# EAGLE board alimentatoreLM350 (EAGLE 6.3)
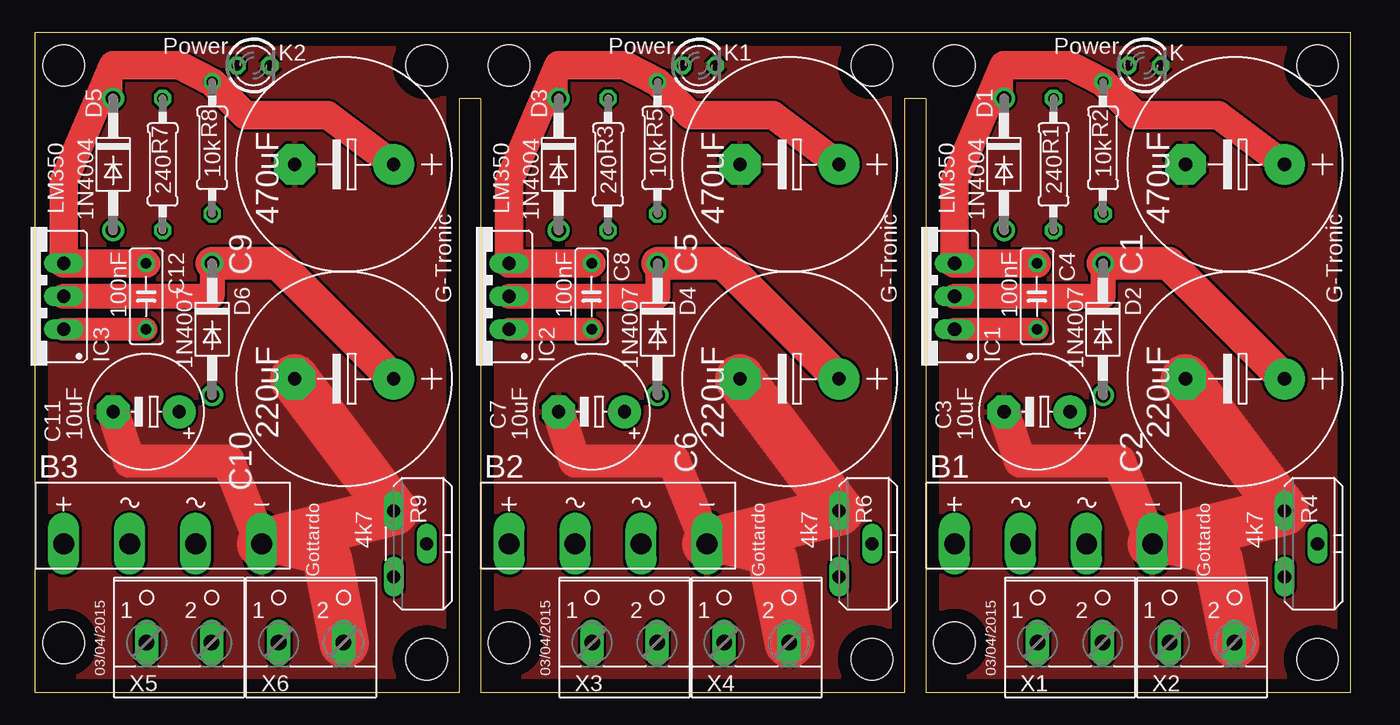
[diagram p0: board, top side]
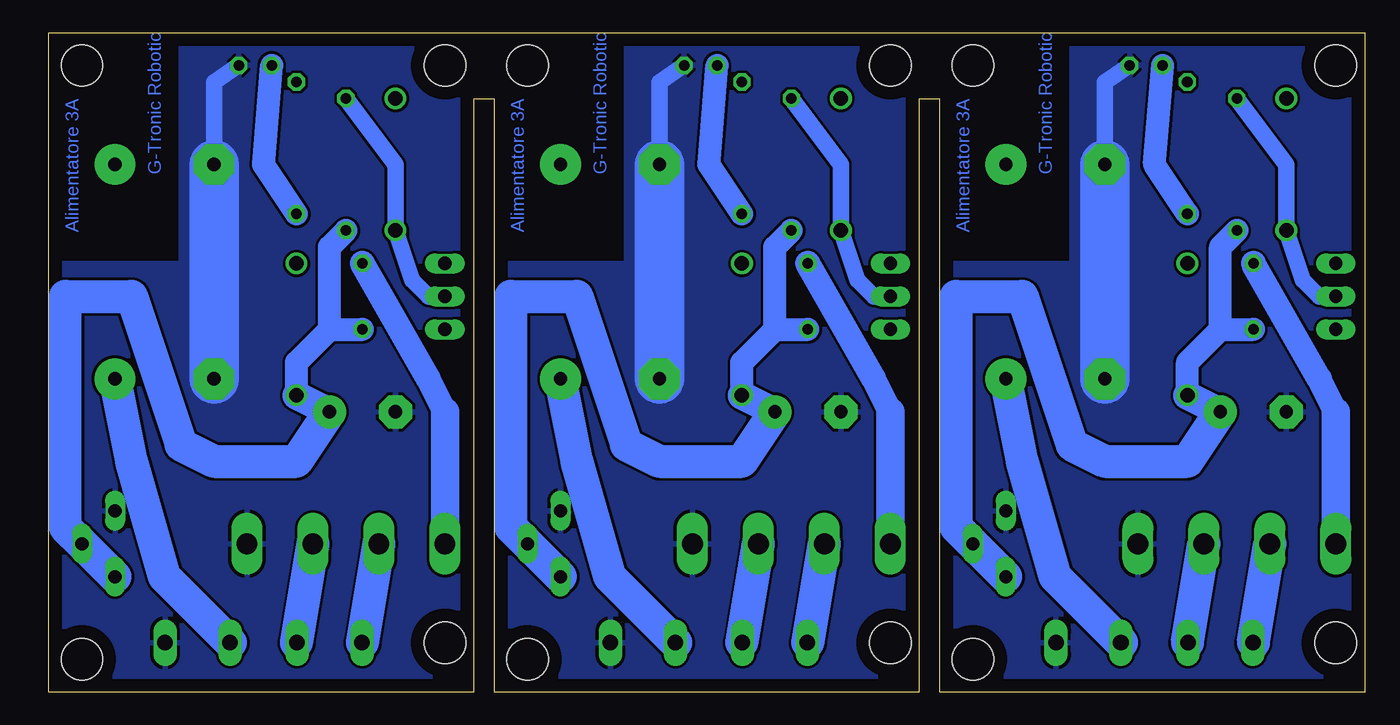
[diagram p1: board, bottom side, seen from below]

Size 101.27 x 50.78 mm. Coordinates in mm from the lower left corner, seen from the top.
Outline: 66.98,50.78 64.44,50.78
Outline: 101.27,0 101.27,50.78 0,50.78 0,0 32.69,0 32.69,45.7 34.29,45.7 34.29,0 66.98,0 66.98,45.7 68.58,45.7 68.58,0 101.27,0
Copper layers (1*16): Top 0.035mm / dielectric 1.5mm / Bottom 0.035mm
Design rules "default": minimum track width 10mil, minimum drill 24mil, track to track 8mil, track to pad 8mil, pad to pad 8mil, via to via 8mil, smd to smd 8mil, copper to edge 40mil, drill to drill 8mil, minimum pad ring 10mil, minimum via ring 8mil, stop-mask expansion 4mil, vias tented up to drill 0mil, thermal gap 10mil
Holes 3.2 mm at 70.79,3.81 98.73,2.54 70.79,48.26 98.73,48.26 36.5,3.81 64.44,2.54 36.5,48.26 64.44,48.26 2.21,3.81 30.15,2.54 2.21,48.26 30.15,48.26

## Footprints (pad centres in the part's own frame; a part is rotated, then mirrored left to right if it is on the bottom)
KBL = drill 1.6 long: + -7.62,-1.27; - 7.62,-1.27; AC1 2.54,-1.27; AC2 -2.54,-1.27
E7,5-16 = drill 1.016 pad 3.15: + -3.81,0 | drill 1.016 pad 3.15 octagon: - 3.81,0
E5-8,5 = drill 1.016 pad 2.54: + -2.54,0 | drill 1.016 pad 2.54 octagon: - 2.54,0
C050-025X075 = drill 0.813 octagon: 1 -2.54,0; 2 2.54,0
DO41-10 = drill 1.118: A 5.08,0; C -5.08,0
317TS = drill 1.016 long: 1 -2.54,-2.54; 2 0,-2.54; 3 2.54,-2.54
LED3MM = drill 0.813 octagon: A -1.27,0; K 1.27,0
0207/10 = drill 0.813 octagon: 1 -5.08,0; 2 5.08,0
PT-10S = drill 1.016 long: A -2.54,-1.27; E 2.54,-1.27; S 0,1.27
W237-102 = drill 1.194 long: 1 -2.5,-1.27; 2 2.5,-1.27

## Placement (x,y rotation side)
B1  [KBL]  78.41,12.7 0 top
B2  [KBL]  44.12,12.7 0 top
B3  [KBL]  9.83,12.7 0 top
C1  470uF  [E7,5-16]  92.38,40.64 180 top
C2  220uF  [E7,5-16]  92.38,24.13 180 top
C3  10uF  [E5-8,5]  77.14,21.59 180 top
C4  100nF  [C050-025X075]  77.14,30.48 270 top
C5  470uF  [E7,5-16]  58.09,40.64 180 top
C6  220uF  [E7,5-16]  58.09,24.13 180 top
C7  10uF  [E5-8,5]  42.85,21.59 180 top
C8  100nF  [C050-025X075]  42.85,30.48 270 top
C9  470uF  [E7,5-16]  23.8,40.64 180 top
C10  220uF  [E7,5-16]  23.8,24.13 180 top
C11  10uF  [E5-8,5]  8.56,21.59 180 top
C12  100nF  [C050-025X075]  8.56,30.48 270 top
D1  1N4004  [DO41-10]  74.6,40.64 270 top
D2  1N4007  [DO41-10]  82.22,27.94 270 top
D3  1N4004  [DO41-10]  40.31,40.64 270 top
D4  1N4007  [DO41-10]  47.93,27.94 270 top
D5  1N4004  [DO41-10]  6.02,40.64 270 top
D6  1N4007  [DO41-10]  13.64,27.94 270 top
IC1  LM350  [317TS]  68.25,30.48 90 top
IC2  LM350  [317TS]  33.96,30.48 90 top
IC3  LM350  [317TS]  -0.33,30.48 90 top
K  Power  [LED3MM]  85.39,48.26 0 top
K1  Power  [LED3MM]  51.11,48.26 0 top
K2  Power  [LED3MM]  16.82,48.26 0 top
R1  240  [0207/10]  78.41,40.64 90 top
R2  10k  [0207/10]  82.22,41.91 90 top
R3  240  [0207/10]  44.12,40.64 90 top
R4  4k7  [PT-10S]  97.46,11.43 270 top
R5  10k  [0207/10]  47.93,41.91 90 top
R6  4k7  [PT-10S]  63.17,11.43 270 top
R7  240  [0207/10]  9.83,40.64 90 top
R8  10k  [0207/10]  13.64,41.91 90 top
R9  4k7  [PT-10S]  28.88,11.43 270 top
X1  [W237-102]  79.68,5.08 0 top
X2  [W237-102]  89.84,5.08 0 top
X3  [W237-102]  45.39,5.08 0 top
X4  [W237-102]  55.55,5.08 0 top
X5  [W237-102]  11.1,5.08 0 top
X6  [W237-102]  21.26,5.08 0 top

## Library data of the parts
B1-B3 = rectifier
C1-C12 R1-R3 R5 R7 R8 = resistor
D1-D6 = diode
IC1-IC3 = v-reg
K K1 K2 = led
R4 R6 R9 = pot
X1-X6 = con-wago-500; MPN: 237-102; OC_FARNELL: unknown; OC_NEWARK: 70K9898

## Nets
GND: B1.- C1.- C2.- C3.- K.K R4.A X2.2
GND1: B2.- C5.- C6.- C7.- K1.K R6.A X4.2
GND2: B3.- C9.- C10.- C11.- K2.K R9.A X6.2
N$1: B1.AC2 X1.1
N$2: B1.AC1 X1.2
N$3: B2.AC2 X3.1
N$4: C3.+ C4.2 D2.A IC1.1 R1.1 R4.E R4.S
N$5: C2.+ D1.A D2.C IC1.2 R1.2 X2.1
N$6: B2.AC1 X3.2
N$7: B1.+ C1.+ C4.1 D1.C IC1.3 R2.2
N$8: K.A R2.1
N$9: C7.+ C8.2 D4.A IC2.1 R3.1 R6.E R6.S
N$10: C6.+ D3.A D4.C IC2.2 R3.2 X4.1
N$11: B2.+ C5.+ C8.1 D3.C IC2.3 R5.2
N$12: K1.A R5.1
N$13: B3.AC2 X5.1
N$14: B3.AC1 X5.2
N$15: C11.+ C12.2 D6.A IC3.1 R7.1 R9.E R9.S
N$16: C10.+ D5.A D6.C IC3.2 R7.2 X6.1
N$17: B3.+ C9.+ C12.1 D5.C IC3.3 R8.2
N$18: K2.A R8.1

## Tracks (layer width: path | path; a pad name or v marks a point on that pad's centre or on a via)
GND
  Top 0.254: X2.2 92.38,3.81
  Top 2.54: 91.11,10.16 B1.- 83.49,17.78 75.87,17.78 C3.-
  Top 3.81: 92.38,3.81 91.11,10.16 | B1.- R4.A C2.-
  Bottom 1.27: K.K 88.57,46.99 C1.-
  Bottom 3.81: C2.- C1.-
  pour Bottom: 68.25,0 68.25,50.8 91.11,50.8 91.11,33.02 101.27,33.02 101.27,0
  pour Top: 68.25,0 68.25,50.8 101.27,50.8 101.27,0
GND1
  Top 0.254: X4.2 58.09,3.81
  Top 2.54: 56.82,10.16 B2.- 49.2,17.78 41.58,17.78 C7.-
  Top 3.81: 58.09,3.81 56.82,10.16 | B2.- R6.A C6.-
  Bottom 1.27: K1.K 54.28,46.99 C5.-
  Bottom 3.81: C6.- C5.-
  pour Bottom: 33.96,0 33.96,50.8 56.82,50.8 56.82,33.02 66.98,33.02 66.98,0
  pour Top: 33.96,0 33.96,50.8 66.98,50.8 66.98,0
GND2
  Top 0.254: X6.2 23.8,3.81
  Top 2.54: 22.53,10.16 B3.- 14.91,17.78 7.29,17.78 C11.-
  Top 3.81: 23.8,3.81 22.53,10.16 | B3.- R9.A C10.-
  Bottom 1.27: K2.K 19.99,46.99 C9.-
  Bottom 3.81: C10.- C9.-
  pour Bottom: -0.33,0 -0.33,50.8 22.53,50.8 22.53,33.02 32.69,33.02 32.69,0
  pour Top: -0.33,0 -0.33,50.8 32.69,50.8 32.69,0
N$1
  Bottom 0.254: X1.1 77.14,3.81
  Bottom 2.54: 77.14,3.81 B1.AC2
N$2
  Bottom 0.254: X1.2 82.22,3.81
  Bottom 2.54: 82.22,3.81 B1.AC1
N$3
  Bottom 0.254: X3.1 42.85,3.81
  Bottom 2.54: 42.85,3.81 B2.AC2
N$4
  Top 1.778: C4.2 IC1.1
  Bottom 1.778: 79.68,27.94 82.22,25.4 D2.A | 79.68,27.94 C4.2 | R1.1 79.68,34.29 79.68,27.94
  Bottom 2.184: C3.+ D2.A
  Bottom 2.54: R4.E R4.S 100,12.7 100,30.48 94.92,30.48 91.11,19.05 88.57,17.78 82.22,17.78 C3.+
N$5
  Top 1.93: D2.C 82.22,30.48 IC1.2
  Top 2.54: C2.+ 87.3,33.02 D2.C
  Bottom 0.254: X2.1 87.3,3.81
  Bottom 1.27: R1.2 74.6,40.64 D1.A 73.33,31.75 72.06,30.48 IC1.2
  Bottom 2.54: 87.3,3.81 92.38,8.89 94.92,17.78 C2.+
N$6
  Bottom 0.254: X3.2 47.93,3.81
  Bottom 2.54: 47.93,3.81 B2.AC1
N$7
  Top 1.422: 74.6,48.26 D1.C
  Top 2.184: C4.1 IC1.3 70.79,39.37 74.6,48.26 79.68,48.26 R2.2 84.76,44.45 91.11,44.45 C1.+
  Bottom 1.93: 70.79,21.59 72.06,24.13 C4.1
  Bottom 2.184: B1.+ 70.79,21.59
N$8
  Bottom 1.778: R2.1 84.76,40.64 K.A
N$9
  Top 1.778: C8.2 IC2.1
  Bottom 1.778: 45.39,27.94 47.93,25.4 D4.A | 45.39,27.94 C8.2 | R3.1 45.39,34.29 45.39,27.94
  Bottom 2.184: C7.+ D4.A
  Bottom 2.54: R6.E R6.S 65.71,12.7 65.71,30.48 60.63,30.48 56.82,19.05 54.28,17.78 47.93,17.78 C7.+
N$10
  Top 1.93: D4.C 47.93,30.48 IC2.2
  Top 2.54: C6.+ 53.01,33.02 D4.C
  Bottom 0.254: X4.1 53.01,3.81
  Bottom 1.27: R3.2 40.31,40.64 D3.A 39.04,31.75 37.77,30.48 IC2.2
  Bottom 2.54: 53.01,3.81 58.09,8.89 60.63,17.78 C6.+
N$11
  Top 1.422: 40.31,48.26 D3.C
  Top 2.184: C8.1 IC2.3 36.5,39.37 40.31,48.26 45.39,48.26 R5.2 50.47,44.45 56.82,44.45 C5.+
  Bottom 1.93: 36.5,21.59 37.77,24.13 C8.1
  Bottom 2.184: B2.+ 36.5,21.59
N$12
  Bottom 1.778: R5.1 50.47,40.64 K1.A
N$13
  Bottom 0.254: X5.1 8.56,3.81
  Bottom 2.54: 8.56,3.81 B3.AC2
N$14
  Bottom 0.254: X5.2 13.64,3.81
  Bottom 2.54: 13.64,3.81 B3.AC1
N$15
  Top 1.778: C12.2 IC3.1
  Bottom 1.778: 11.1,27.94 13.64,25.4 D6.A | 11.1,27.94 C12.2 | R7.1 11.1,34.29 11.1,27.94
  Bottom 2.184: C11.+ D6.A
  Bottom 2.54: R9.E R9.S 31.42,12.7 31.42,30.48 26.34,30.48 22.53,19.05 19.99,17.78 13.64,17.78 C11.+
N$16
  Top 1.93: D6.C 13.64,30.48 IC3.2
  Top 2.54: C10.+ 18.72,33.02 D6.C
  Bottom 0.254: X6.1 18.72,3.81
  Bottom 1.27: R7.2 6.02,40.64 D5.A 4.75,31.75 3.48,30.48 IC3.2
  Bottom 2.54: 18.72,3.81 23.8,8.89 26.34,17.78 C10.+
N$17
  Top 1.422: 6.02,48.26 D5.C
  Top 2.184: C12.1 IC3.3 2.21,39.37 6.02,48.26 11.1,48.26 R8.2 16.18,44.45 22.53,44.45 C9.+
  Bottom 1.93: 2.21,21.59 3.48,24.13 C12.1
  Bottom 2.184: B3.+ 2.21,21.59
N$18
  Bottom 1.778: R8.1 16.18,40.64 K2.A

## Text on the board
Bottom: G-Tronic Robotic | G-Tronic Robotic | G-Tronic Robotic | Alimentatore 3A | Alimentatore 3A | Alimentatore 3A
tNames: G-Tronic | G-Tronic | G-Tronic | Gottardo | Gottardo | Gottardo | 03/04/2015 | 03/04/2015 | 03/04/2015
